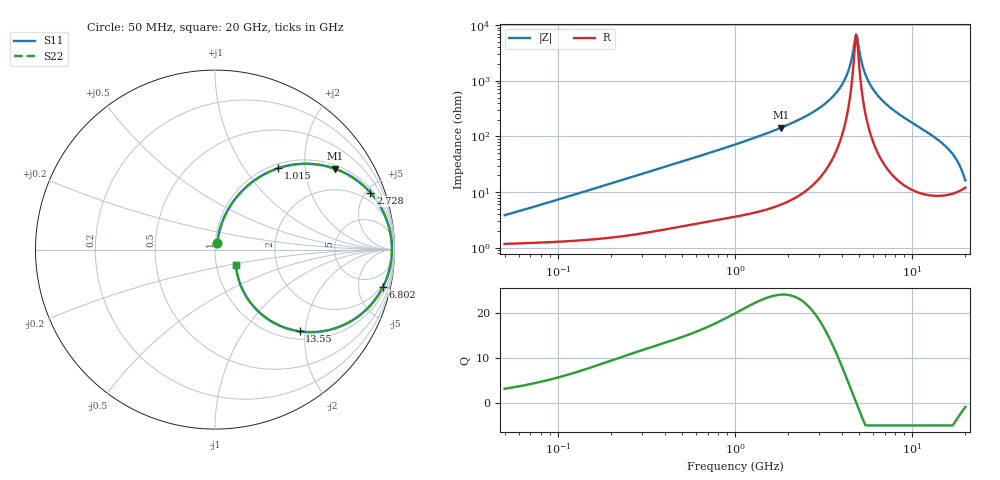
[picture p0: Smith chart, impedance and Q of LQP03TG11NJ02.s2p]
!Murata Part Number: LQP03TG11NJ02
!These Parameters are Measured in Series Mode Connection
!  o--[Z]--o
!Port1  Port2
!  o-------o
!Freq. Start=50[MHz] Stop=20[GHz], 401[Steps]
# Hz S RI R 50
!Freq.(Hz) S11(Real) S11(Imag) S21(Real) S21(Imag) S12(Real) S12(Imag) S22(Real) S22(Imag)
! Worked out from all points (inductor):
!   401 points, 50 MHz to 20 GHz, reference 50 ohm
!   read as one part in series: L = 11.6 nH near 51.52 MHz
!   highest Q = 24 at 1.821 GHz (marker M1), where L = 12.5 nH
!   self-resonance near 4.82 GHz
!   S11 on the Smith chart (normalised r, x): 50 MHz: 1.02, +0.07; 1.015 GHz: 1.07, +1.45; 2.728 GHz: 1.26, +5.36; 6.802 GHz: 1.70, -8.78; 13.55 GHz: 1.17, -1.87; 20 GHz: 1.24, -0.22
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5e7  0.0129 0.0358  0.9871 -0.0358  0.9871 -0.0358  0.0129 0.0358
1.364002e8  0.0226 0.0947  0.9774 -0.0947  0.9774 -0.0947  0.0226 0.0947
3.721004e8  0.0814 0.2374  0.9186 -0.2374  0.9186 -0.2374  0.0814 0.2374
6.285508e8  0.1795 0.3539  0.8205 -0.3539  0.8205 -0.3539  0.1795 0.3539
1e9  0.3461 0.4512  0.6539 -0.4512  0.6539 -0.4512  0.3461 0.4512
1.015091e9  0.353 0.4535  0.647 -0.4535  0.647 -0.4535  0.353 0.4535
1.820564e9  0.6666 0.451  0.3334 -0.451  0.3334 -0.451  0.6666 0.451
2.728004e9  0.8662 0.3169  0.1338 -0.3169  0.1338 -0.3169  0.8662 0.3169
3.415248e9  0.9405 0.2042  0.0595 -0.2042  0.0595 -0.2042  0.9405 0.2042
3.967106e9  0.971 0.1195  0.029 -0.1195  0.029 -0.1195  0.971 0.1195
4.34015e9  0.9814 0.0663  0.0186 -0.0663  0.0186 -0.0663  0.9814 0.0663
4.748272e9  0.9856 0.0118  0.0144 -0.0118  0.0144 -0.0118  0.9856 0.0118
4.81993e9  0.9857 0.00266  0.0143 -0.00266  0.0143 -0.00266  0.9857 0.00266
4.966507e9  0.9854 -0.0157  0.0146 0.0157  0.0146 0.0157  0.9854 -0.0157
5.273168e9  0.9825 -0.0526  0.0175 0.0526  0.0175 0.0526  0.9825 -0.0526
5.598765e9  0.9766 -0.0896  0.0234 0.0896  0.0234 0.0896  0.9766 -0.0896
6.802353e9  0.9359 -0.2081  0.0641 0.2081  0.0641 0.2081  0.9359 -0.2081
7.442007e9  0.9051 -0.2605  0.0949 0.2605  0.0949 0.2605  0.9051 -0.2605
1.050288e10  0.7066 -0.4244  0.2934 0.4244  0.2934 0.4244  0.7066 -0.4244
1.354865e10  0.4719 -0.4555  0.5281 0.4555  0.5281 0.4555  0.4719 -0.4555
1.696185e10  0.2294 -0.3326  0.7706 0.3326  0.7706 0.3326  0.2294 -0.3326
2e10  0.116 -0.0855  0.884 0.0855  0.884 0.0855  0.116 -0.0855
